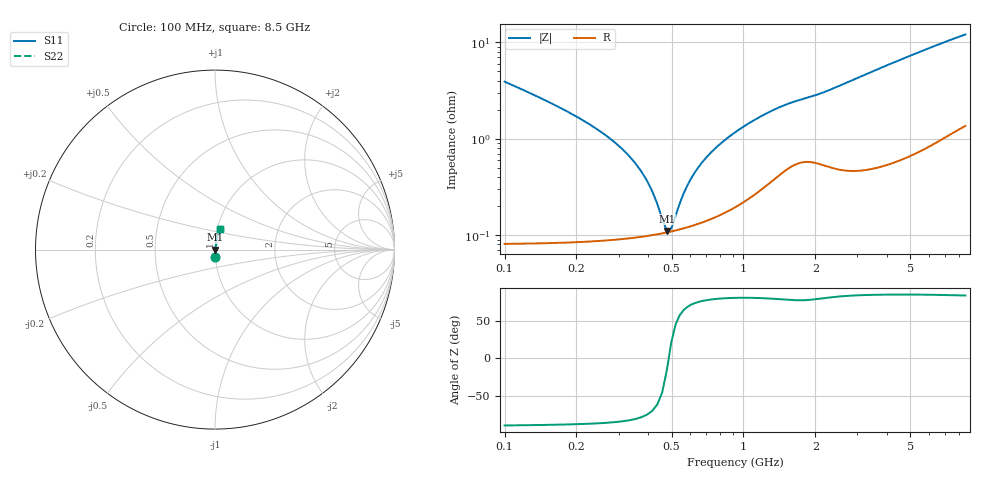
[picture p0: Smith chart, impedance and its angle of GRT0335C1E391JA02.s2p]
!Murata Part Number: GRT0335C1E391JA02
!These Parameters are Measured in Series Mode Connection
!Data Generated on Jun 19, 2026
!  o--ll--o
!Port1  Port2
!  o------o
!Operation Temp=25[degC], DC Bias Voltage=0[V]
!Freq. Start=100[MHz] Stop=9[GHz] 401[Steps]
# Hz S RI R 50
!Freq.(Hz) S11(Real) S11(Imag) S21(Real) S21(Imag) S12(Real) S12(Imag) S22(Real) S22(Imag)
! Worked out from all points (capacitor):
!   401 points, 100 MHz to 8.5 GHz, reference 50 ohm
!   read as one part in series: C = 390 pF near 142 MHz
!   lowest |Z| = 110 mohm at 478 MHz (marker M1)
!   series resonance near 486.4 MHz, so ESL is about 270 pH
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1e8  0.00233 -0.039  0.9977 0.039  0.9977 0.039  0.00233 -0.039
1.42e8  0.00151 -0.0262  0.9985 0.0262  0.9985 0.0262  0.00151 -0.0262
3.31e8  0.000967 -0.00661  0.999 0.00661  0.999 0.00661  0.000967 -0.00661
3.94e8  0.00099 -0.00355  0.999 0.00355  0.999 0.00355  0.00099 -0.00355
4.36e8  0.00102 -0.00183  0.999 0.00183  0.999 0.00183  0.00102 -0.00183
4.57e8  0.00104 -0.00104  0.999 0.00104  0.999 0.00104  0.00104 -0.00104
4.78e8  0.00107 -0.000288  0.9989 0.000288  0.9989 0.000288  0.00107 -0.000288
4.99e8  0.00109 0.000432  0.9989 -0.000432  0.9989 -0.000432  0.00109 0.000432
5.2e8  0.00112 0.00112  0.9989 -0.00112  0.9989 -0.00112  0.00112 0.00112
5.83e8  0.00121 0.00306  0.9988 -0.00306  0.9988 -0.00306  0.00121 0.00306
6.46e8  0.00133 0.00482  0.9987 -0.00482  0.9987 -0.00482  0.00133 0.00482
7.09e8  0.00146 0.00646  0.9985 -0.00646  0.9985 -0.00646  0.00146 0.00646
7.93e8  0.00167 0.00851  0.9983 -0.00851  0.9983 -0.00851  0.00167 0.00851
9.19e8  0.00206 0.0114  0.9979 -0.0114  0.9979 -0.0114  0.00206 0.0114
1.087e9  0.00273 0.0149  0.9973 -0.0149  0.9973 -0.0149  0.00273 0.0149
1.297e9  0.00386 0.0187  0.9961 -0.0187  0.9961 -0.0187  0.00386 0.0187
1.507e9  0.00518 0.0219  0.9948 -0.0219  0.9948 -0.0219  0.00518 0.0219
2.914e9  0.00627 0.0407  0.9937 -0.0407  0.9937 -0.0407  0.00627 0.0407
4.3e9  0.00943 0.0612  0.9906 -0.0612  0.9906 -0.0612  0.00943 0.0612
5.707e9  0.0143 0.0808  0.9857 -0.0808  0.9857 -0.0808  0.0143 0.0808
7.114e9  0.0204 0.099  0.9796 -0.099  0.9796 -0.099  0.0204 0.099
8.5e9  0.027 0.1151  0.973 -0.1151  0.973 -0.1151  0.027 0.1151
